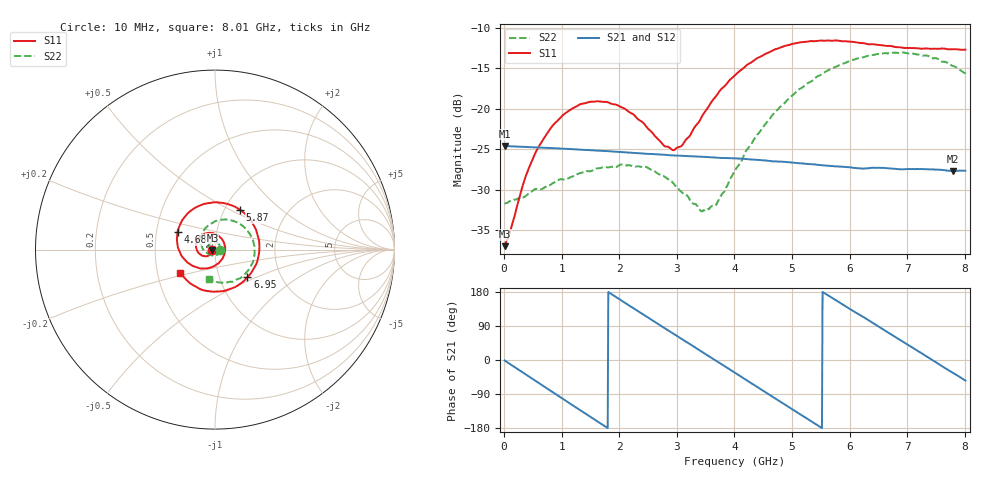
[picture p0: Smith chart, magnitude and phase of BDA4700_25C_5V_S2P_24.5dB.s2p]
!Agilent Technologies,E5071B,MY42404982,A.09.10
!Date: Mon Oct 20 13:38:47 2025
!Data & Calibration Information:
!Freq	S11:SOLT2(ON)	S21:SOLT2(ON)	S12:SOLT2(ON)	S22:SOLT2(ON)
# Hz S RI R 50
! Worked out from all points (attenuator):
!   801 points, 10 MHz to 8.01 GHz, reference 50 ohm
!   highest |S21| = -24.58 dB at 20 MHz (marker M1); lowest = -27.7 dB at 7.79 GHz (marker M2)
!   lowest |S11| = -37.0 dB at 10 MHz (marker M3), VSWR 1.03, Z = 48.6 - j0.142 ohm
!   |S11| at or under -10 dB: start of sweep to end of sweep
!   |S22| runs from -32.7 to -13.0 dB; largest |S21 - S12| = 0.0005
!   S11 on the Smith chart (normalised r, x): 10 MHz: 0.97, -0.00; 4.68 GHz: 0.64, +0.13; 5.87 GHz: 1.17, +0.56; 6.95 GHz: 1.36, -0.44; 8.01 GHz: 0.66, -0.18
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1e7  -0.0141 -0.00146  0.059 -0.00128  0.059 -0.00135  0.0261 -0.000806
2e7  -0.0145 -0.00226  0.059 -0.00226  0.059 -0.00241  0.026 -0.00109
3.6e8  -0.0255 -0.0266  0.0466 -0.0347  0.0467 -0.0347  0.022 -0.0184
5.8e8  -0.0432 -0.0365  0.03 -0.0493  0.03 -0.0493  0.014 -0.0286
9.9e8  -0.0856 -0.0243  -0.00935 -0.056  -0.00937 -0.0561  -0.0141 -0.0338
1.35e9  -0.1061 0.0165  -0.0397 -0.0394  -0.0397 -0.0394  -0.0361 -0.0178
1.99e9  -0.0525 0.09  -0.0514 0.017  -0.0515 0.017  -0.0335 0.0295
2.68e9  0.0476 0.0438  -0.00413 0.0521  -0.00415 0.0521  0.013 0.0373
2.92e9  0.0557 -0.000345  0.0165 0.0488  0.0165 0.0488  0.0247 0.0252
3.06e9  0.0511 -0.0282  0.0273 0.0434  0.0271 0.0435  0.0275 0.0146
3.44e9  -0.0018 -0.0903  0.0471 0.0183  0.0472 0.0183  0.0185 -0.0141
3.69e9  -0.059 -0.1053  0.0499 -0.00246  0.0499 -0.0026  0.000405 -0.0257
4.01e9  -0.1387 -0.0818  0.0411 -0.0275  0.0411 -0.0274  -0.0325 -0.0258
4.68e9  -0.2089 0.0984  -0.00721 -0.0468  -0.00714 -0.0468  -0.0799 0.0481
5.35e9  -0.0515 0.2565  -0.0436 -0.0131  -0.0435 -0.0132  -0.0154 0.1481
5.87e9  0.1376 0.2221  -0.0369 0.0237  -0.0369 0.0236  0.1006 0.1605
6.26e9  0.2304 0.1049  -0.0157 0.0398  -0.0154 0.0398  0.1816 0.1035
6.68e9  0.2367 -0.0614  0.0137 0.0406  0.0138 0.0406  0.2202 -3.28e-05
6.95e9  0.1805 -0.1537  0.0292 0.0306  0.0294 0.0305  0.2099 -0.0733
7.36e9  0.0362 -0.2324  0.042 0.00531  0.042 0.00525  0.1385 -0.1608
7.79e9  -0.1324 -0.1922  0.0343 -0.0228  0.0343 -0.0229  0.0224 -0.1827
8.01e9  -0.1922 -0.1299  0.0242 -0.0337  0.0243 -0.0337  -0.0309 -0.1618
